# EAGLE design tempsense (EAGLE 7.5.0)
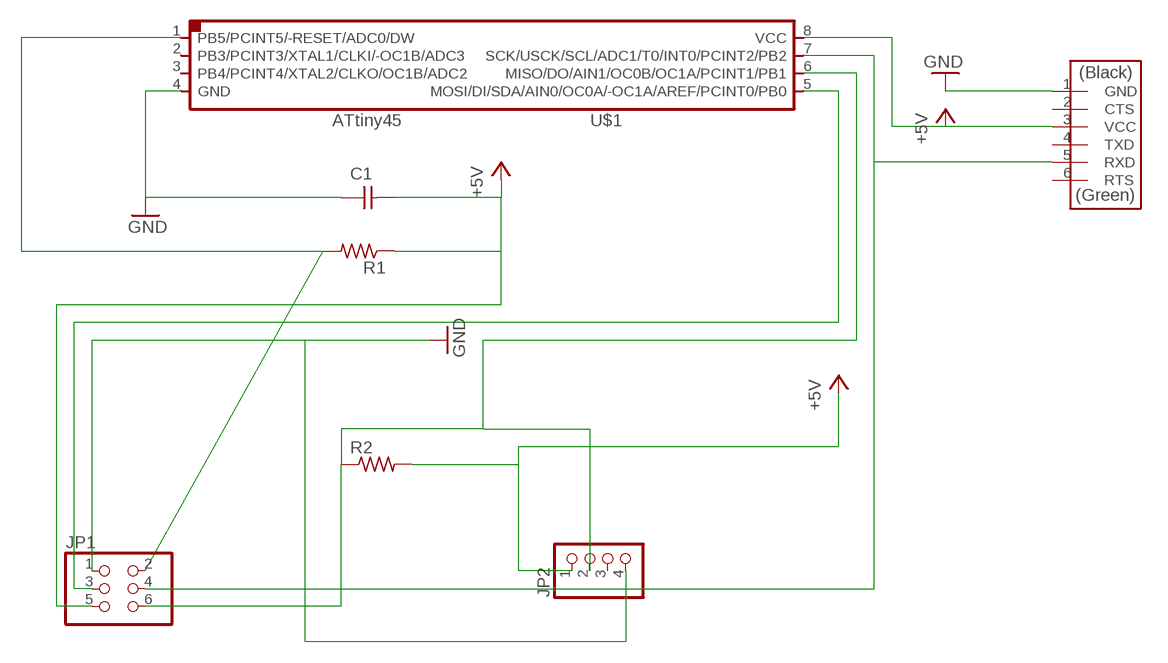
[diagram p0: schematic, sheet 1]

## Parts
C1  CAP-UNPOLARIZEDFAB  [C1206FAB]
JP1  PINHD-2X3-SMD  [2X03SMD]
JP2  PINHD-1X4  [1X04]
R1  RES-US1206FAB  [R1206FAB]
R2  RES-US1206FAB  [R1206FAB]
U$1  ATTINY45SI  [SOIC8]
U$2  FTDI-SMD-HEADER  [1X06SMD]

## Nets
+5V: C1.2 JP1.5 JP2.1 R1.1 R2.2 U$1.8(VCC) U$2.3(VCC)
GND: C1.1 JP1.1 JP2.4 U$1.4(GND) U$2.1(GND)
N$2: JP1.4 U$1.7(SCK/USCK/SCL/ADC1/T0/INT0/PCINT2/PB2) U$2.5(RXD)
N$3: JP1.2 R1.2 U$1.1(PB5/PCINT5/-RESET/ADC0/DW)
N$4: JP1.3 U$1.5(MOSI/DI/SDA/AIN0/OC0A/-OC1A/AREF/PCINT0/PB0)
N$7: JP1.6 JP2.2 R2.1 U$1.6(MISO/DO/AIN1/OC0B/OC1A/PCINT1/PB1)
Unconnected: JP2.3 U$1.2(PB3/PCINT3/XTAL1/CLKI/-OC1B/ADC3) U$1.3(PB4/PCINT4/XTAL2/CLKO/OC1B/ADC2) U$2.2(CTS) U$2.4(TXD) U$2.6(RTS)

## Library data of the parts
C1 = fab:CAP-UNPOLARIZED
JP1 = fab:PINHD-2X3-SMD: PIN HEADER
JP2 = pinhead:PINHD-1X4: PIN HEADER
R1 R2 = fab:RES-US: Resistor (US Symbol)
U$1 = fab:ATTINY45
U$2 = fab:FTDI-SMD-HEADER

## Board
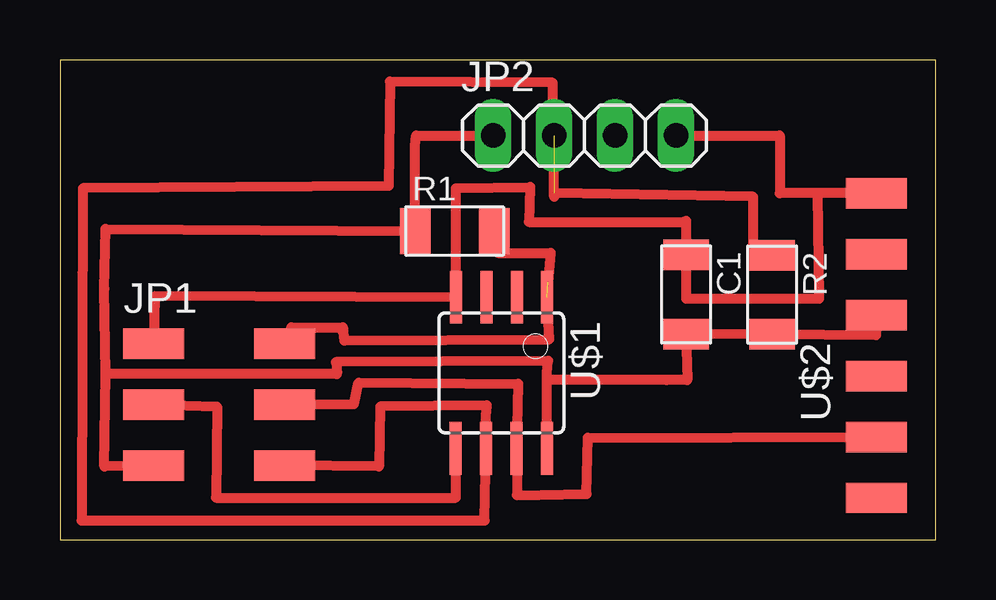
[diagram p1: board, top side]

Size 36.5 x 20 mm. Coordinates in mm from the lower left corner, seen from the top.
Outline: 0,0 36.5,0 36.5,20 0,20 0,0
Copper layers 1: Top 0.035mm
Design rules "default *": minimum track width 10mil, minimum drill 24mil, track to track 0.42mm, track to pad 0.42mm, pad to pad 8mil, via to via 8mil, smd to smd 8mil, copper to edge 1mil, drill to drill 8mil, minimum pad ring 10mil, minimum via ring 8mil, stop-mask expansion 4mil, vias tented up to drill 0mil, thermal gap 10mil

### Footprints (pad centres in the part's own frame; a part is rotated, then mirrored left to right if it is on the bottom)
C1206FAB = smd 1.27 x 1.905: 1 -1.651,0; 2 1.651,0
2X03SMD = smd 2.54 x 1.27: 1 -2.54,2.54; 2 2.92,2.54; 3 -2.54,0; 4 2.92,0; 5 -2.54,-2.54; 6 2.92,-2.54
1X04 = drill 1.016 long: 1 -3.81,0; 2 -1.27,0; 3 1.27,0; 4 3.81,0
R1206FAB = smd 1.27 x 1.905: 1 -1.651,0; 2 1.651,0
SOIC8 = smd 0.5 x 2.2: 1 -1.905,-3.154; 2 -0.645,-3.154; 3 0.625,-3.154; 4 1.895,-3.154; 5 1.905,3.154; 6 0.635,3.154; 7 -0.635,3.154; 8 -1.905,3.154
1X06SMD = smd 2.54 x 1.27: 1 0,6.35; 2 0,3.81; 3 0,1.27; 4 0,-1.27; 5 0,-3.81; 6 0,-6.35

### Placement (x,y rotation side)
C1  26.1,10.22 270 top
JP1  6.45,5.63 0 top
JP2  21.87,16.85 0 top
R1  16.46,12.86 0 top
R2  29.69,10.21 270 top
U$1  18.4,6.95 180 top
U$2  34.03,8.09 0 top

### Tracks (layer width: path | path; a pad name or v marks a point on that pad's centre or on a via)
+5V
  Top 0.406: U$2.3 34.03,8.52 R2.2 C1.2 26.15,6.65 25.3,6.65 20.3,6.65 | JP1.5 1.85,3.05 1.9,6.9 | 1.9,6.9 1.85,10.45 1.9,12.95 R1.1 14.8,16.4 14.85,16.85 JP2.1 | U$1.8 20.3,6.65 | 20.3,6.65 20.3,6.95 20.35,7.45 11.5,7.4 11.55,6.9 1.9,6.9
GND
  Top 0.406: U$2.1 31.6,14.44 | 31.6,14.44 30,14.44 30,16.85 JP2.4 | 31.6,14.44 31.65,10.05 26.1,10.05 C1.1 26.1,13.3 26,13.25 19.55,13.25 19.6,14.7 16.5,14.65 U$1.4 3.95,10.15 JP1.1
N$2
  Top 0.406: U$2.5 22,4.25 21.95,1.9 19.05,1.85 U$1.7 19.1,6.5 12.45,6.55 12.25,5.65 JP1.4
N$3  (1 unrouted)
  Top 0.406: R1.2 18.25,11.95 20.45,11.95 20.35,10.75 | JP1.2 9.65,8.85 11.8,8.85 11.8,8.65 11.85,8.3 20.4,8.35 U$1.1
N$4
  Top 0.406: JP1.3 6.55,5.55 6.5,1.75 16.5,1.75 U$1.5
N$7  (1 unrouted)
  Top 0.406: R2.1 28.9,11.85 28.9,14.3 20.6,14.45 20.6,14.3 20.55,19.05 13.75,19.1 13.7,14.75 0.95,14.65 0.9,0.8 17.7,0.8 U$1.6 17.75,5.15 17.8,5.6 13.35,5.55 13.3,3.05 JP1.6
